| z11b_ver7.ibs * IBIS 5.0 Model
| Part Number   VDD/VDDQ   Architecture   Package
| MT40A1G8SA   1.2V/1.2V   1Gb   x 8   78-Ball FBGA
[IBIS Ver]   7.0
[File Name]   z11b_ver7.ibs
[Date]   04/03/2019
[File Rev]   1.0
[Source]   From silicon level SPICE model at Micron Technology, Inc.
[Notes]   Revision History:
   Rev 1.0: 04/03/2019
   - Initial IBIS Version 7.0 model
   - Includes Interconnect Model examples
   - Unofficial IBIS model for syntax evaluation purposes.
[Disclaimer]  This software code and all associated documentation, comments
   or other information (collectively "Software") is provided
   "AS IS" without warranty of any kind. MICRON TECHNOLOGY, INC.
   ("MTI") EXPRESSLY DISCLAIMS ALL WARRANTIES EXPRESS OR IMPLIED,
   INCLUDING BUT NOT LIMITED TO, NONINFRINGEMENT OF THIRD PARTY
   RIGHTS, AND ANY IMPLIED WARRANTIES OF MERCHANTABILITY OR
   FITNESS FOR ANY PARTICULAR PURPOSE. MTI DOES NOT WARRANT THAT
   THE SOFTWARE WILL MEET YOUR REQUIREMENTS, OR THAT THE
   OPERATION OF THE SOFTWARE WILL BE UNINTERRUPTED OR ERROR-FREE.
   FURTHERMORE, MTI DOES NOT MAKE ANY REPRESENTATIONS REGARDING
   THE USE OR THE RESULTS OF THE USE OF THE SOFTWARE IN TERMS OF
   ITS CORRECTNESS, ACCURACY, RELIABILITY, OR OTHERWISE. THE
   ENTIRE RISK ARISING OUT OF USE OR PERFORMANCE OF THE SOFTWARE
   REMAINS WITH YOU. IN NO EVENT SHALL MTI, ITS AFFILIATED
   COMPANIES OR THEIR SUPPLIERS BE LIABLE FOR ANY DIRECT,
   INDIRECT, CONSEQUENTIAL, INCIDENTAL, OR SPECIAL DAMAGES
   (INCLUDING, WITHOUT LIMITATION, DAMAGES FOR LOSS OF PROFITS,
   BUSINESS INTERRUPTION, OR LOSS OF INFORMATION) ARISING OUT OF
   YOUR USE OF OR INABILITY TO USE THE SOFTWARE, EVEN IF MTI HAS
   BEEN ADVISED OF THE POSSIBILITY OF SUCH DAMAGES. Because some
   jurisdictions prohibit the exclusion or limitation of
   liability for consequential or incidental damages, the above
   limitation may not apply to you.
   Additional Disclaimer:
   This IBIS model is unoffical and is provided to the IBIS Open
   Forum for the purposes of evaluating the IBIS Version 7.0
   syntax.  This model is not intended to accurately represent
   the characteristics of any official product.
[Copyright]   Copyright 2019 Micron Technology, Inc. All rights reserved.
| COMPONENT: MT40A1G8SA (78-Ball FBGA, x8)
[Component]   MT40A1G8SA
[Package Model] z11b_78ball_pkg
[Manufacturer]  Micron Technology,Inc.
[Package]
|   typ   min   max
R_pkg   0.420   0.337   0.508
L_pkg   1.872nH   1.600nH   2.256nH
C_pkg   0.503pF   0.373pF   0.869pF
[Pin]   signal_name   model_name   R_pin   L_pin   C_pin   | TD_pin(ps)   Z_pin
A1   VDD   POWER
A2   VSS   GND
A3   TDQS_c   TDQS   0.462   1.686nH   0.497pF   |  28.960   58.214
A7   DM_n_DBI_n_TDQS_t   DM_DBI_TDQS   0.471   1.769nH   0.574pF   |  31.858   55.533
A8   VSS   GND
A9   VSS   GND
B1   VPP   POWER
B2   VDDQ   POWER
B3   DQS_c   DQS   0.477   1.698nH   0.518pF   |  29.650   57.266
B7   DQ1   DQ   0.462   1.634nH   0.572pF   |  30.578   53.451
B8   VDDQ   POWER
B9   ZQ   NC   0.508   2.256nH   0.824pF   |  43.107   52.342
C1   VDDQ   POWER
C2   DQ0   DQ   0.462   1.655nH   0.561pF   |  30.473   54.297
C3   DQS_t   DQS   0.474   1.833nH   0.464pF   |  29.170   62.828
C7   VDD   POWER
C8   VSS   GND
C9   VDDQ   POWER
D1   VSS   GND
D2   DQ4   DQ   0.480   1.664nH   0.568pF   |  30.747   54.122
D3   DQ2   DQ   0.467   1.763nH   0.499pF   |  29.645   59.463
D7   DQ3   DQ   0.459   1.706nH   0.562pF   |  30.957   55.111
D8   DQ5   DQ   0.462   1.600nH   0.541pF   |  29.424   54.382
D9   VSS   GND
E1   VSSL   GND
E2   VDDQ   POWER
E3   DQ6   DQ   0.464   1.695nH   0.554pF   |  30.652   55.303
E7   DQ7   DQ   0.467   1.715nH   0.555pF   |  30.855   55.582
E8   VDDQ   POWER
E9   VSS   GND
F1   VDDL   POWER
F2   NC   NC
F3   ODT   INPUT   0.416   2.081nH   0.465pF   |  31.112   66.890
F7   CK_t   CLKIN   0.415   1.748nH   0.464pF   |  28.489   61.372
F8   CK_c   CLKIN   0.410   1.679nH   0.519pF   |  29.522   56.862
F9   VDD   POWER
G1   VSS   GND
G2   NC   NC
G3   CKE   INPUT   0.408   2.148nH   0.421pF   |  30.082   71.417
G7   CS_n   INPUT   0.410   1.936nH   0.441pF   |  29.202   66.289
G8   NC   NC
G9   TEN   TEN   0.391   2.104nH   0.869pF   |  42.760   49.210
H1   VDD   POWER
H2   WE_n_A14   INPUT   0.399   2.037nH   0.466pF   |  30.823   66.098
H3   ACT_n   INPUT   0.402   1.924nH   0.413pF   |  28.187   68.247
H7   CAS_n_A15   INPUT   0.400   1.971nH   0.388pF   |  27.650   71.272
H8   RAS_n   INPUT   0.402   1.982nH   0.473pF   |  30.603   64.755
H9   VSS   GND
J1   VREFCA   POWER
J2   BG0   INPUT   0.401   1.934nH   0.446pF   |  29.359   65.889
J3   A10   INPUT   0.401   1.866nH   0.389pF   |  26.938   69.285
J7   A12_BC_n   INPUT   0.399   1.954nH   0.373pF   |  26.994   72.369
J8   BG1   INPUT   0.404   2.030nH   0.462pF   |  30.632   66.264
J9   VDD   POWER
K1   VSS   GND
K2   BA0   INPUT   0.400   1.977nH   0.479pF   |  30.781   64.232
K3   A4   INPUT   0.400   1.907nH   0.431pF   |  28.681   66.498
K7   A3   INPUT   0.401   1.966nH   0.421pF   |  28.788   68.301
K8   BA1   INPUT   0.400   2.056nH   0.465pF   |  30.918   66.499
K9   VSS   GND
L1   RESET_n   RESET   0.341   1.708nH   0.725pF   |  35.193   48.541
L2   A6   INPUT   0.400   1.879nH   0.480pF   |  30.031   62.571
L3   A0   INPUT   0.401   1.714nH   0.418pF   |  26.769   64.010
L7   A1   INPUT   0.406   1.901nH   0.423pF   |  28.361   67.015
L8   A5   INPUT   0.405   1.943nH   0.492pF   |  30.910   62.868
L9   ALERT_n   ALERT   0.337   1.799nH   0.707pF   |  35.671   50.442
M1   VDD   POWER
M2   A8   INPUT   0.401   1.929nH   0.476pF   |  30.313   63.619
M3   A2   INPUT   0.403   1.906nH   0.404pF   |  27.738   68.700
M7   A9   INPUT   0.405   1.974nH   0.395pF   |  27.924   70.677
M8   A7   INPUT   0.402   2.015nH   0.488pF   |  31.361   64.239
M9   VPP   POWER
N1   VSS   GND
N2   A11   INPUT   0.401   1.858nH   0.497pF   |  30.379   61.148
N3   PARITY   INPUT   0.402   1.724nH   0.471pF   |  28.492   60.493
N7   NC   NC
N8   A13   INPUT   0.404   2.043nH   0.479pF   |  31.277   65.327
N9   VDD   POWER
|***********************PIN MAPPING*****************************************
[Pin Mapping]   pulldown_ref   pullup_ref   gnd_clamp_ref   power_clamp_ref ext_ref
A1   NC   VDD
A2   VSS   NC
A3   VSS   VDDQ   VSS   VDDQ
A7   VSS   VDDQ   VSS   VDDQ
A8   VSS   NC
A9   VSS   NC
B1   NC   VPP
B2   NC   VDDQ
B3   VSS   VDDQ   VSS   VDDQ
B7   VSS   VDDQ   VSS   VDDQ
B8   NC   VDDQ
B9   NC   NC
C1   NC   VDDQ
C2   VSS   VDDQ   VSS   VDDQ
C3   VSS   VDDQ   VSS   VDDQ
C7   NC   VDD
C8   VSS   NC
C9   NC   VDDQ
D1   VSS   NC
D2   VSS   VDDQ   VSS   VDDQ
D3   VSS   VDDQ   VSS   VDDQ
D7   VSS   VDDQ   VSS   VDDQ
D8   VSS   VDDQ   VSS   VDDQ
D9   VSS   NC
E1   VSSL   NC
E2   NC   VDDQ
E3   VSS   VDDQ   VSS   VDDQ
E7   VSS   VDDQ   VSS   VDDQ
E8   NC   VDDQ
E9   VSS   NC
F1   NC   VDDL
F2   NC   NC
F3   NC   NC   VSS   VDD
F7   NC   NC   VSS   VDD
F8   NC   NC   VSS   VDD
F9   NC   VDD
G1   VSS   NC
G2   NC   NC
G3   NC   NC   VSS   VDD
G7   NC   NC   VSS   VDD
G8   NC   NC
G9   NC   NC   VSS   VDD
H1   NC   VDD
H2   NC   NC   VSS   VDD
H3   NC   NC   VSS   VDD
H7   NC   NC   VSS   VDD
H8   NC   NC   VSS   VDD
H9   VSS   NC
J1   NC   VREFCA
J2   NC   NC   VSS   VDD
J3   NC   NC   VSS   VDD
J7   NC   NC   VSS   VDD
J8   NC   NC   VSS   VDD
J9   NC   VDD
K1   VSS   NC
K2   NC   NC   VSS   VDD
K3   NC   NC   VSS   VDD
K7   NC   NC   VSS   VDD
K8   NC   NC   VSS   VDD
K9   VSS   NC
L1   NC   NC   VSS   VDD
L2   NC   NC   VSS   VDD
L3   NC   NC   VSS   VDD
L7   NC   NC   VSS   VDD
L8   NC   NC   VSS   VDD
L9   VSS   VDDQ   VSS   VDDQ
M1   NC   VDD
M2   NC   NC   VSS   VDD
M3   NC   NC   VSS   VDD
M7   NC   NC   VSS   VDD
M8   NC   NC   VSS   VDD
M9   NC   VPP
N1   VSS   NC
N2   NC   NC   VSS   VDD
N3   NC   NC   VSS   VDD
N7   NC   NC
N8   NC   NC   VSS   VDD
N9   NC   VDD
|**********************DIE SUPPLY PADS**************************************
[Die Supply Pads]  signal_name   bus_label
VDDQ_DIE-4   VDDQ
VDDQ_DIE-8   VDDQ
VDDQ_DIE-13   VDDQ
VDDQ_DIE-16   VDDQ
VDDQ_DIE-20   VDDQ
VDDQ_DIE-25   VDDQ
VDDQ_DIE-36   VDDQ
VDDQ_DIE-48   VDDQ
VDDQ_DIE-52   VDDQ
VDDQ_DIE-62   VDDQ
VDDQ_DIE-40   VDDQ
VDDQ_DIE-45   VDDQ
VDDQ_DIE-57   VDDQ
VSS_DIE-2   VSS
VSS_DIE-6   VSS
VSS_DIE-10   VSS
VSS_DIE-11   VSS
VSS_DIE-15   VSS
VSS_DIE-18   VSS
VSS_DIE-22   VSS
VSS_DIE-23   VSS
VSS_DIE-27   VSS
VSS_DIE-28   VSS
VSS_DIE-32   VSS
VSS_DIE-34   VSS
VSS_DIE-38   VSS
VSS_DIE-42   VSS
VSS_DIE-43   VSS
VSS_DIE-47   VSS
VSS_DIE-50   VSS
VSS_DIE-54   VSS
VSS_DIE-55   VSS
VSS_DIE-59   VSS
VSS_DIE-60   VSS
VSS_DIE-64   VSS
VSS_DIE-66   VSS
VSS_DIE-69   VSS
VSS_DIE-72   VSS
VSS_DIE-93   VSS
VSS_DIE-109   VSS
VSS_DIE-117   VSS
|**********************DIFF PIN*********************************************
[Diff_pin]   inv_pin   vdiff   tdelay_typ   tdelay_min   tdelay_max
   C3   B3   0.000V   0ns   NA   NA
   F7   F8   0.250V   0ns   NA   NA
|**********************INTERCONNECT MODEL GROUPS****************************
| Interconnect Model Group for MT40A1G8SA_DQ_Signal_ISS
| Device:   MT40A1G8SA
| Signals:  DQ, DQS, DM
| Coupling: Yes
| PDN:   Ideal
| Decap:   None
| Type:   Quasi-static Spice Model
[Interconnect Model Group]  MT40A1G8SA_DQ_Signal_ISS
| Interconnect Model Set   file_reference
MT40A1G8SA_DQ_Signal_ISS   NA
[End Interconnect Model Group]
| Interconnect Model Group for MT40A1G8SA_CA_Signal_ISS
| Device:   MT40A1G8SA
| Signals:  Add, Cmd, Ctl, CLK
| Coupling: Yes
| PDN:   Ideal
| Decap:   None
| Type:   Quasi-static Spice Model
[Interconnect Model Group]  MT40A1G8SA_CA_Signal_ISS
| Interconnect Model Set   file_reference
MT40A1G8SA_CA_Signal_ISS   NA
[End Interconnect Model Group]
| Interconnect Model Group for MT40A1G8SA_Full_Pkg_ISS
| Device:   MT40A1G8SA
| Signals:  All
| Coupling: Yes
| PDN:   Package Parasitics
| Decap:   On-die
| Type:   Quasi-static Spice Model
[Interconnect Model Group]  MT40A1G8SA_Full_Pkg_ISS
| Interconnect Model Set   file_reference
MT40A1G8SA_Full_Pkg_ISS   NA
OnDie_Decoupling_AllDQ   NA
[End Interconnect Model Group]
| Interconnect Model Group for MT40A1G8SA_DQ_Signal_BB_ISS
| Device:   MT40A1G8SA
| Signals:  DQ, DQS, DM
| Coupling: Yes
| PDN:   Reference
| Decap:   None
| Type:   Full-wave Spice Model
[Interconnect Model Group]  MT40A1G8SA_DQ_Signal_BB_ISS
| Interconnect Model Set   file_reference
MT40A1G8SA_DQ_Signal_BB_ISS   NA
[End Interconnect Model Group]
| Interconnect Model Group for MT40A1G8SA_DQ_Signal_Sparam
| Device:   MT40A1G8SA
| Signals:  DQ, DQS, DM
| Coupling: Yes
| PDN:   Reference
| Decap:   None
| Type:   Full-wave S-parameter Model
[Interconnect Model Group]  MT40A1G8SA_DQ_Signal_Sparam
| Interconnect Model Set   file_reference
MT40A1G8SA_DQ_Signal_Sparam   NA
[End Interconnect Model Group]
| Interconnect Model Group for MT40A1G8SA_DQ_TS2_Sparam
| Device:   MT40A1G8SA
| Signals:  DQ, DQS, DM
| Coupling: Yes
| PDN:   Package Parasitics
| Decap:   On-die
| Type:   Full-wave S-parameter Touchstone 2.0 Model
[Interconnect Model Group]  MT40A1G8SA_DQ_TS2_Sparam
| Interconnect Model Set   file_reference
MT40A1G8SA_DQ_TS2_Sparam   NA
OnDie_Decoupling_AllDQ   NA
[End Interconnect Model Group]
| Interconnect Model Group for MT40A1G8SA_DQ_Pkg_Plus_Ondie_PDN_ISS
| Device:   MT40A1G8SA
| Signals:  DQ, DQS, DM
| Coupling: Yes
| PDN:   Package Parasitics, On-die Parasitics
| Decap:   On-die
| Type:   Quasi-static Spice Model + On-die PDN Spice Model
[Interconnect Model Group]  MT40A1G8SA_DQ_Pkg_Plus_Ondie_PDN_ISS
| Interconnect Model Set   file_reference
MT40A1G8SA_DQ_Pkg_Plus_Ondie_PDN_ISS   NA
[End Interconnect Model Group]
| Interconnect Model Group for MT40A1G8SA_DQ_Uncoupled_Sparam
| Device:   MT40A1G8SA
| Signals:  DQ, DQS, DM
| Coupling: No
| PDN:   Reference
| Decap:   On-die
| Type:   Full-wave S-parameter Models
[Interconnect Model Group]  MT40A1G8SA_DQ_Uncoupled_Sparam
| Interconnect Model Set   file_reference
MT40A1G8SA_DQ_Uncoupled_Sparam   NA
[End Interconnect Model Group]
|   Model Selector
[Model Selector] DQ
DQ_34_3200   34 Ohm Data I/O with no ODT, 1600-3200Mbps
DQ_40_3200   40 Ohm Data I/O with no ODT, 1600-3200Mbps
DQ_48_3200   48 Ohm Data I/O with no ODT, 1600-3200Mbps
DQ_IN_ODTOFF_3200  Data Input with no ODT, 1600-3200Mbps
DQ_IN_ODT34_3200   Data Input with 34ohm ODT, 1600-3200Mbps
DQ_IN_ODT40_3200   Data Input with 40ohm ODT, 1600-3200Mbps
DQ_IN_ODT48_3200   Data Input with 48ohm ODT, 1600-3200Mbps
DQ_IN_ODT60_3200   Data Input with 60ohm ODT, 1600-3200Mbps
DQ_IN_ODT80_3200   Data Input with 80ohm ODT, 1600-3200Mbps
DQ_IN_ODT120_3200  Data Input with 120ohm ODT, 1600-3200Mbps
DQ_IN_ODT240_3200  Data Input with 240ohm ODT, 1600-3200Mbps
[Model Selector] DQS
DQS_34_3200   34 Ohm Data Strobe I/O with no ODT, 1600-3200Mbps
DQS_40_3200   40 Ohm Data Strobe I/O with no ODT, 1600-3200Mbps
DQS_48_3200   48 Ohm Data Strobe I/O with no ODT, 1600-3200Mbps
DQS_IN_ODTOFF_3200 Data Strobe Input with no ODT, 1600-3200Mbps
DQS_IN_ODT34_3200  Data Strobe Input with 34ohm ODT, 1600-3200Mbps
DQS_IN_ODT40_3200  Data Strobe Input with 40ohm ODT, 1600-3200Mbps
DQS_IN_ODT48_3200  Data Strobe Input with 48ohm ODT, 1600-3200Mbps
DQS_IN_ODT60_3200  Data Strobe Input with 60ohm ODT, 1600-3200Mbps
DQS_IN_ODT80_3200  Data Strobe Input with 80ohm ODT, 1600-3200Mbps
DQS_IN_ODT120_3200 Data Strobe Input with 120ohm ODT, 1600-3200Mbps
DQS_IN_ODT240_3200 Data Strobe Input with 240ohm ODT, 1600-3200Mbps
[Model Selector] DM_DBI
DM_ODTOFF_3200   DM Input Model with no ODT, 1600-3200Mbps
DM_ODT34_3200   DM Input Model with 34ohm ODT, 1600-3200Mbps
DM_ODT40_3200   DM Input Model with 40ohm ODT, 1600-3200Mbps
DM_ODT48_3200   DM Input Model with 48ohm ODT, 1600-3200Mbps
DM_ODT60_3200   DM Input Model with 60ohm ODT, 1600-3200Mbps
DM_ODT80_3200   DM Input Model with 80ohm ODT, 1600-3200Mbps
DM_ODT120_3200   DM Input Model with 120ohm ODT, 1600-3200Mbps
DM_ODT240_3200   DM Input Model with 240ohm ODT, 1600-3200Mbps
DQ_34_3200   34 Ohm DBI I/O with no ODT, 1600-3200Mbps
DQ_40_3200   40 Ohm DBI I/O with no ODT, 1600-3200Mbps
DQ_48_3200   48 Ohm DBI I/O with no ODT, 1600-3200Mbps
DQ_IN_ODTOFF_3200  DBI Input with no ODT, 1600-3200Mbps
DQ_IN_ODT34_3200   DBI Input with 34ohm ODT, 1600-3200Mbps
DQ_IN_ODT40_3200   DBI Input with 40ohm ODT, 1600-3200Mbps
DQ_IN_ODT48_3200   DBI Input with 48ohm ODT, 1600-3200Mbps
DQ_IN_ODT60_3200   DBI Input with 60ohm ODT, 1600-3200Mbps
DQ_IN_ODT80_3200   DBI Input with 80ohm ODT, 1600-3200Mbps
DQ_IN_ODT120_3200  DBI Input with 120ohm ODT, 1600-3200Mbps
DQ_IN_ODT240_3200  DBI Input with 240ohm ODT, 1600-3200Mbps
NF_DQ   Non-Functioning DQ Terminator Model
[Model Selector] DM_DBI_TDQS
DM_ODTOFF_3200   DM Input Model with no ODT, 1600-3200Mbps
DM_ODT34_3200   DM Input Model with 34ohm ODT, 1600-3200Mbps
DM_ODT40_3200   DM Input Model with 40ohm ODT, 1600-3200Mbps
DM_ODT48_3200   DM Input Model with 48ohm ODT, 1600-3200Mbps
DM_ODT60_3200   DM Input Model with 60ohm ODT, 1600-3200Mbps
DM_ODT80_3200   DM Input Model with 80ohm ODT, 1600-3200Mbps
DM_ODT120_3200   DM Input Model with 120ohm ODT, 1600-3200Mbps
DM_ODT240_3200   DM Input Model with 240ohm ODT, 1600-3200Mbps
DQ_34_3200   34 Ohm DBI I/O with no ODT, 1600-3200Mbps
DQ_40_3200   40 Ohm DBI I/O with no ODT, 1600-3200Mbps
DQ_48_3200   48 Ohm DBI I/O with no ODT, 1600-3200Mbps
DQ_IN_ODTOFF_3200  DBI Input with no ODT, 1600-3200Mbps
DQ_IN_ODT34_3200   DBI Input with 34ohm ODT, 1600-3200Mbps
DQ_IN_ODT40_3200   DBI Input with 40ohm ODT, 1600-3200Mbps
DQ_IN_ODT48_3200   DBI Input with 48ohm ODT, 1600-3200Mbps
DQ_IN_ODT60_3200   DBI Input with 60ohm ODT, 1600-3200Mbps
DQ_IN_ODT80_3200   DBI Input with 80ohm ODT, 1600-3200Mbps
DQ_IN_ODT120_3200  DBI Input with 120ohm ODT, 1600-3200Mbps
DQ_IN_ODT240_3200  DBI Input with 240ohm ODT, 1600-3200Mbps
TDQS_ODTOFF_3200   TDQS Terminator Model with no ODT, 1600-3200Mbps
TDQS_ODT34_3200   TDQS Terminator Model with 34ohm ODT, 1600-3200Mbps
TDQS_ODT40_3200   TDQS Terminator Model with 40ohm ODT, 1600-3200Mbps
TDQS_ODT48_3200   TDQS Terminator Model with 48ohm ODT, 1600-3200Mbps
TDQS_ODT60_3200   TDQS Terminator Model with 60ohm ODT, 1600-3200Mbps
TDQS_ODT80_3200   TDQS Terminator Model with 80ohm ODT, 1600-3200Mbps
TDQS_ODT120_3200   TDQS Terminator Model with 120ohm ODT, 1600-3200Mbps
TDQS_ODT240_3200   TDQS Terminator Model with 240ohm ODT, 1600-3200Mbps
NF_DQ   Non-Functioning DQ Terminator Model
[Model Selector] TDQS
TDQS_ODTOFF_3200   TDQS Terminator Model with no ODT, 1600-3200Mbps
TDQS_ODT34_3200   TDQS Terminator Model with 34ohm ODT, 1600-3200Mbps
TDQS_ODT40_3200   TDQS Terminator Model with 40ohm ODT, 1600-3200Mbps
TDQS_ODT48_3200   TDQS Terminator Model with 48ohm ODT, 1600-3200Mbps
TDQS_ODT60_3200   TDQS Terminator Model with 60ohm ODT, 1600-3200Mbps
TDQS_ODT80_3200   TDQS Terminator Model with 80ohm ODT, 1600-3200Mbps
TDQS_ODT120_3200   TDQS Terminator Model with 120ohm ODT, 1600-3200Mbps
TDQS_ODT240_3200   TDQS Terminator Model with 240ohm ODT, 1600-3200Mbps
NF_DQ   Non-Functioning DQ Terminator Model
| Sparse Matrix Package Model for z11b_78ball_pkg (x4/x8)
[Define Package Model]  z11b_78ball_pkg
[Manufacturer]   Micron Technology, Inc.
[OEM]   Micron Technology, Inc.
[Description]   z11b package model for 78-ball x4/x8 FBGA
[Number of Pins]   51
[Pin Numbers]
L3  | A0
L7  | A1
M3  | A2
K7  | A3
K3  | A4
L8  | A5
L2  | A6
M8  | A7
M2  | A8
M7  | A9
J3  | A10
N2  | A11
J7  | A12
N8  | A13
H3  | ACT#
L9  | ALERT#
K2  | BA0
K8  | BA1
J2  | BG0
J8  | BG1
H7  | CAS#
G3  | CKE
F8  | CK_C
F7  | CK_T
G7  | CS#
F3  | ODT
N3  | PARITY
H8  | RAS#
L1  | RESET#
H2  | WE#
C2  | DQ0
D3  | DQ2
D2  | DQ4
E3  | DQ6
B3  | DQS-C
C3  | DQS-T
A3  | TDQS-C
A7  | DM#
B7  | DQ1
D7  | DQ3
D8  | DQ5
E7  | DQ7
G9  | TEN
A1  | VDD
B2  | VDDQ_SUBNET_0
B8  | VDDQ_SUBNET_1
B1  | VPP-B1
M9  | VPP-M9
J1  | VREFCA
A9  | VSS
B9  | ZQ
[Model Data]
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[End Model Data]
[End Package Model]
| Interconnect Model Set for MT40A1G8SA_DQ_Signal_ISS
[Interconnect Model Set]   MT40A1G8SA_DQ_Signal_ISS
[Manufacturer]   Micron Technology, Inc.
[Description]   Z11B 78b, DQ signal only, Coupled Spice Package Model
[Interconnect Model]   z11b_78b_pkg_dq_iss
File_IBIS-ISS   z11b_78b_pkg_dq.iss   z11b_rlc_dq_pkg
Number_of_terminals = 25
1   Buffer_I/O   pin_name   A7   |   DM_n_DBI_n_TDQS_t  DM_DBI_TDQS
2   Buffer_I/O   pin_name   C2   |   DQ0   DQ
3   Buffer_I/O   pin_name   B7   |   DQ1   DQ
4   Buffer_I/O   pin_name   D3   |   DQ2   DQ
5   Buffer_I/O   pin_name   D7   |   DQ3   DQ
6   Buffer_I/O   pin_name   D2   |   DQ4   DQ
7   Buffer_I/O   pin_name   D8   |   DQ5   DQ
8   Buffer_I/O   pin_name   E3   |   DQ6   DQ
9   Buffer_I/O   pin_name   E7   |   DQ7   DQ
10   Buffer_I/O   pin_name   B3   |   DQS_c   DQS
11   Buffer_I/O   pin_name   C3   |   DQS_t   DQS
12   Buffer_I/O   pin_name   A3   |   TDQS_c   TDQS
13   Pin_I/O   pin_name   A7   |   DM_n_DBI_n_TDQS_t  DM_DBI_TDQS
14   Pin_I/O   pin_name   C2   |   DQ0   DQ
15   Pin_I/O   pin_name   B7   |   DQ1   DQ
16   Pin_I/O   pin_name   D3   |   DQ2   DQ
17   Pin_I/O   pin_name   D7   |   DQ3   DQ
18   Pin_I/O   pin_name   D2   |   DQ4   DQ
19   Pin_I/O   pin_name   D8   |   DQ5   DQ
20   Pin_I/O   pin_name   E3   |   DQ6   DQ
21   Pin_I/O   pin_name   E7   |   DQ7   DQ
22   Pin_I/O   pin_name   B3   |   DQS_c   DQS
23   Pin_I/O   pin_name   C3   |   DQS_t   DQS
24   Pin_I/O   pin_name   A3   |   TDQS_c   TDQS
25   Pin_Rail   signal_name   VSS   |   VSS   GND
[End Interconnect Model]
[End Interconnect Model Set]
| Interconnect Model Set for MT40A1G8SA_CA_Signal_ISS
[Interconnect Model Set]   MT40A1G8SA_CA_Signal_ISS
[Manufacturer]   Micron Technology, Inc.
[Description]   Z11B 78b, CA signal only, Coupled Spice Package Model
[Interconnect Model]   z11b_78b_pkg_ca_iss
File_IBIS-ISS   z11b_78b_pkg_ca.iss   z11b_rlc_ca_pkg
Number_of_terminals = 63
1   Buffer_I/O   pin_name   L3   |   A0   INPUT
2   Buffer_I/O   pin_name   L7   |   A1   INPUT
3   Buffer_I/O   pin_name   M3   |   A2   INPUT
4   Buffer_I/O   pin_name   K7   |   A3   INPUT
5   Buffer_I/O   pin_name   K3   |   A4   INPUT
6   Buffer_I/O   pin_name   L8   |   A5   INPUT
7   Buffer_I/O   pin_name   L2   |   A6   INPUT
8   Buffer_I/O   pin_name   M8   |   A7   INPUT
9   Buffer_I/O   pin_name   M2   |   A8   INPUT
10   Buffer_I/O   pin_name   M7   |   A9   INPUT
11   Buffer_I/O   pin_name   J3   |   A10   INPUT
12   Buffer_I/O   pin_name   N2   |   A11   INPUT
13   Buffer_I/O   pin_name   J7   |   A12_BC_n   INPUT
14   Buffer_I/O   pin_name   N8   |   A13   INPUT
15   Buffer_I/O   pin_name   H3   |   ACT_n   INPUT
16   Buffer_I/O   pin_name   L9   |   ALERT_n   ALERT
17   Buffer_I/O   pin_name   K2   |   BA0   INPUT
18   Buffer_I/O   pin_name   K8   |   BA1   INPUT
19   Buffer_I/O   pin_name   J2   |   BG0   INPUT
20   Buffer_I/O   pin_name   J8   |   BG1   INPUT
21   Buffer_I/O   pin_name   H7   |   CAS_n_A15   INPUT
22   Buffer_I/O   pin_name   G3   |   CKE   INPUT
23   Buffer_I/O   pin_name   F8   |   CK_c   CLKIN
24   Buffer_I/O   pin_name   F7   |   CK_t   CLKIN
25   Buffer_I/O   pin_name   G7   |   CS_n   INPUT
26   Buffer_I/O   pin_name   N3   |   PARITY   INPUT
27   Buffer_I/O   pin_name   H8   |   RAS_n   INPUT
28   Buffer_I/O   pin_name   L1   |   RESET_n   RESET
29   Buffer_I/O   pin_name   G9   |   TEN   TEN
30   Buffer_Rail   bus_label   VREFCA  |   VREFCA   POWER
31   Buffer_I/O   pin_name   H2   |   WE_n_A14   INPUT
32   Pin_I/O   pin_name   L3   |   A0   INPUT
33   Pin_I/O   pin_name   L7   |   A1   INPUT
34   Pin_I/O   pin_name   M3   |   A2   INPUT
35   Pin_I/O   pin_name   K7   |   A3   INPUT
36   Pin_I/O   pin_name   K3   |   A4   INPUT
37   Pin_I/O   pin_name   L8   |   A5   INPUT
38   Pin_I/O   pin_name   L2   |   A6   INPUT
39   Pin_I/O   pin_name   M8   |   A7   INPUT
40   Pin_I/O   pin_name   M2   |   A8   INPUT
41   Pin_I/O   pin_name   M7   |   A9   INPUT
42   Pin_I/O   pin_name   J3   |   A10   INPUT
43   Pin_I/O   pin_name   N2   |   A11   INPUT
44   Pin_I/O   pin_name   J7   |   A12_BC_n   INPUT
45   Pin_I/O   pin_name   N8   |   A13   INPUT
46   Pin_I/O   pin_name   H3   |   ACT_n   INPUT
47   Pin_I/O   pin_name   L9   |   ALERT_n   ALERT
48   Pin_I/O   pin_name   K2   |   BA0   INPUT
49   Pin_I/O   pin_name   K8   |   BA1   INPUT
50   Pin_I/O   pin_name   J2   |   BG0   INPUT
51   Pin_I/O   pin_name   J8   |   BG1   INPUT
52   Pin_I/O   pin_name   H7   |   CAS_n_A15   INPUT
53   Pin_I/O   pin_name   G3   |   CKE   INPUT
54   Pin_I/O   pin_name   F8   |   CK_c   CLKIN
55   Pin_I/O   pin_name   F7   |   CK_t   CLKIN
56   Pin_I/O   pin_name   G7   |   CS_n   INPUT
57   Pin_I/O   pin_name   N3   |   PARITY   INPUT
58   Pin_I/O   pin_name   H8   |   RAS_n   INPUT
59   Pin_I/O   pin_name   L1   |   RESET_n   RESET
60   Pin_I/O   pin_name   G9   |   TEN   TEN
61   Pin_Rail   pin_name   J1   |   VREFCA   POWER
62   Pin_I/O   pin_name   H2   |   WE_n_A14   INPUT
63   Pin_Rail   signal_name   VSS   |   VSS   GND
[End Interconnect Model]
[End Interconnect Model Set]
| Interconnect Model Set for MT40A1G8SA_Full_Pkg_ISS
[Interconnect Model Set]   MT40A1G8SA_Full_Pkg_ISS
[Manufacturer]   Micron Technology, Inc.
[Description]   Z11B 78b, Full Package, Coupled Spice Model
[Interconnect Model]   z11b_78b_full_pkg_iss
File_IBIS-ISS   z11b_78b_full_pkg.iss   z11b_rlc_all_pkg
Number_of_terminals = 104
1   Buffer_I/O   pin_name   L3   |   A0   INPUT
2   Buffer_I/O   pin_name   L7   |   A1   INPUT
3   Buffer_I/O   pin_name   M3   |   A2   INPUT
4   Buffer_I/O   pin_name   K7   |   A3   INPUT
5   Buffer_I/O   pin_name   K3   |   A4   INPUT
6   Buffer_I/O   pin_name   L8   |   A5   INPUT
7   Buffer_I/O   pin_name   L2   |   A6   INPUT
8   Buffer_I/O   pin_name   M8   |   A7   INPUT
9   Buffer_I/O   pin_name   M2   |   A8   INPUT
10   Buffer_I/O   pin_name   M7   |   A9   INPUT
11   Buffer_I/O   pin_name   J3   |   A10   INPUT
12   Buffer_I/O   pin_name   N2   |   A11   INPUT
13   Buffer_I/O   pin_name   J7   |   A12_BC_n   INPUT
14   Buffer_I/O   pin_name   N8   |   A13   INPUT
15   Buffer_I/O   pin_name   H3   |   ACT_n   INPUT
16   Buffer_I/O   pin_name   L9   |   ALERT_n   ALERT
17   Buffer_I/O   pin_name   K2   |   BA0   INPUT
18   Buffer_I/O   pin_name   K8   |   BA1   INPUT
19   Buffer_I/O   pin_name   J2   |   BG0   INPUT
20   Buffer_I/O   pin_name   J8   |   BG1   INPUT
21   Buffer_I/O   pin_name   H7   |   CAS_n_A15   INPUT
22   Buffer_I/O   pin_name   G3   |   CKE   INPUT
23   Buffer_I/O   pin_name   F8   |   CK_c   CLKIN
24   Buffer_I/O   pin_name   F7   |   CK_t   CLKIN
25   Buffer_I/O   pin_name   G7   |   CS_n   INPUT
26   Buffer_I/O   pin_name   A7   |   DM_n_DBI_n_TDQS_t  DM_DBI_TDQS
27   Buffer_I/O   pin_name   C2   |   DQ0   DQ
28   Buffer_I/O   pin_name   B7   |   DQ1   DQ
29   Buffer_I/O   pin_name   D3   |   DQ2   DQ
30   Buffer_I/O   pin_name   D7   |   DQ3   DQ
31   Buffer_I/O   pin_name   D2   |   DQ4   DQ
32   Buffer_I/O   pin_name   D8   |   DQ5   DQ
33   Buffer_I/O   pin_name   E3   |   DQ6   DQ
34   Buffer_I/O   pin_name   E7   |   DQ7   DQ
35   Buffer_I/O   pin_name   B3   |   DQS_c   DQS
36   Buffer_I/O   pin_name   C3   |   DQS_t   DQS
37   Buffer_I/O   pin_name   F3   |   ODT   INPUT
38   Buffer_I/O   pin_name   N3   |   PARITY   INPUT
39   Buffer_I/O   pin_name   H8   |   RAS_n   INPUT
40   Buffer_I/O   pin_name   L1   |   RESET_n   RESET
41   Buffer_I/O   pin_name   A3   |   TDQS_c   TDQS
42   Buffer_I/O   pin_name   G9   |   TEN   TEN
43   Buffer_Rail   bus_label   VDD   |   VDD   POWER
44   Buffer_Rail   bus_label   VDDL   |   VDDL   POWER
45   Buffer_Rail   bus_label   VDDQ   |   VDDQ   POWER
46   Buffer_Rail   bus_label   VDDQ   |   VDDQ   POWER
47   Buffer_Rail   bus_label   VPP   |   VPP   POWER
48   Buffer_Rail   bus_label   VPP   |   VPP   POWER
49   Buffer_Rail   bus_label   VREFCA  |   VREFCA   POWER
50   Buffer_Rail   bus_label   VSS   |   VSS   GND
51   Buffer_I/O   pin_name   H2   |   WE_n_A14   INPUT
52   Buffer_I/O   pin_name   B9   |   ZQ   NC
53   Pin_I/O   pin_name   L3   |   A0   INPUT
54   Pin_I/O   pin_name   L7   |   A1   INPUT
55   Pin_I/O   pin_name   M3   |   A2   INPUT
56   Pin_I/O   pin_name   K7   |   A3   INPUT
57   Pin_I/O   pin_name   K3   |   A4   INPUT
58   Pin_I/O   pin_name   L8   |   A5   INPUT
59   Pin_I/O   pin_name   L2   |   A6   INPUT
60   Pin_I/O   pin_name   M8   |   A7   INPUT
61   Pin_I/O   pin_name   M2   |   A8   INPUT
62   Pin_I/O   pin_name   M7   |   A9   INPUT
63   Pin_I/O   pin_name   J3   |   A10   INPUT
64   Pin_I/O   pin_name   N2   |   A11   INPUT
65   Pin_I/O   pin_name   J7   |   A12_BC_n   INPUT
66   Pin_I/O   pin_name   N8   |   A13   INPUT
67   Pin_I/O   pin_name   H3   |   ACT_n   INPUT
68   Pin_I/O   pin_name   L9   |   ALERT_n   ALERT
69   Pin_I/O   pin_name   K2   |   BA0   INPUT
70   Pin_I/O   pin_name   K8   |   BA1   INPUT
71   Pin_I/O   pin_name   J2   |   BG0   INPUT
72   Pin_I/O   pin_name   J8   |   BG1   INPUT
73   Pin_I/O   pin_name   H7   |   CAS_n_A15   INPUT
74   Pin_I/O   pin_name   G3   |   CKE   INPUT
75   Pin_I/O   pin_name   F8   |   CK_c   CLKIN
76   Pin_I/O   pin_name   F7   |   CK_t   CLKIN
77   Pin_I/O   pin_name   G7   |   CS_n   INPUT
78   Pin_I/O   pin_name   A7   |   DM_n_DBI_n_TDQS_t  DM_DBI_TDQS
79   Pin_I/O   pin_name   C2   |   DQ0   DQ
80   Pin_I/O   pin_name   B7   |   DQ1   DQ
81   Pin_I/O   pin_name   D3   |   DQ2   DQ
82   Pin_I/O   pin_name   D7   |   DQ3   DQ
83   Pin_I/O   pin_name   D2   |   DQ4   DQ
84   Pin_I/O   pin_name   D8   |   DQ5   DQ
85   Pin_I/O   pin_name   E3   |   DQ6   DQ
86   Pin_I/O   pin_name   E7   |   DQ7   DQ
87   Pin_I/O   pin_name   B3   |   DQS_c   DQS
88   Pin_I/O   pin_name   C3   |   DQS_t   DQS
89   Pin_I/O   pin_name   F3   |   ODT   INPUT
90   Pin_I/O   pin_name   N3   |   PARITY   INPUT
91   Pin_I/O   pin_name   H8   |   RAS_n   INPUT
92   Pin_I/O   pin_name   L1   |   RESET_n   RESET
93   Pin_I/O   pin_name   A3   |   TDQS_c   TDQS
94   Pin_I/O   pin_name   G9   |   TEN   TEN
95   Pin_Rail   pin_name   A1   |   VDD   POWER
96   Pin_Rail   pin_name   F1   |   VDDL   POWER
97   Pin_Rail   pin_name   B2   |   VDDQ   POWER
98   Pin_Rail   pin_name   C9   |   VDDQ   POWER
99   Pin_Rail   pin_name   B1   |   VPP   POWER
100   Pin_Rail   pin_name   M9   |   VPP   POWER
101   Pin_Rail   pin_name   J1   |   VREFCA   POWER
102   Pin_Rail   pin_name   A9   |   VSS   GND
103   Pin_I/O   pin_name   H2   |   WE_n_A14   INPUT
104   Pin_I/O   pin_name   B9   |   ZQ   NC
[End Interconnect Model]
[End Interconnect Model Set]
| Interconnect Model Set for OnDie_Decoupling_AllDQ
[Interconnect Model Set]   OnDie_Decoupling_AllDQ
[Interconnect Model]   z11b_ondie_decoupling_alldq_iss
File_IBIS-ISS   z11b_ondie_decoupling_alldq.iss   z11b_ondie_decoupling_alldq
Number_of_terminals = 4
1   Buffer_Rail   bus_label   VDDQ   |   VDDQ   POWER
2   Buffer_Rail   bus_label   VDD   |   VDD   POWER
3   Buffer_Rail   bus_label   VSS   |   VSS   GND
4   A_gnd
[End Interconnect Model]
[End Interconnect Model Set]
| Interconnect Model Set for MT40A1G8SA_DQ_Signal_BB_ISS
[Interconnect Model Set]   MT40A1G8SA_DQ_Signal_BB_ISS
[Interconnect Model]   z11b_78b_bb_dq_pkg_iss
File_IBIS-ISS   z11b_78b_bb_dq_pkg.iss   z11b_bb_dq_pkg
Number_of_terminals = 25
1   Pin_I/O   pin_name   A7   |   DM_n_DBI_n_TDQS_t  DM_DBI_TDQS
2   Buffer_I/O   pin_name   A7   |   DM_n_DBI_n_TDQS_t  DM_DBI_TDQS
3   Pin_I/O   pin_name   C2   |   DQ0   DQ
4   Buffer_I/O   pin_name   C2   |   DQ0   DQ
5   Pin_I/O   pin_name   B7   |   DQ1   DQ
6   Buffer_I/O   pin_name   B7   |   DQ1   DQ
7   Pin_I/O   pin_name   D3   |   DQ2   DQ
8   Buffer_I/O   pin_name   D3   |   DQ2   DQ
9   Pin_I/O   pin_name   D7   |   DQ3   DQ
10   Buffer_I/O   pin_name   D7   |   DQ3   DQ
11   Pin_I/O   pin_name   D2   |   DQ4   DQ
12   Buffer_I/O   pin_name   D2   |   DQ4   DQ
13   Pin_I/O   pin_name   D8   |   DQ5   DQ
14   Buffer_I/O   pin_name   D8   |   DQ5   DQ
15   Pin_I/O   pin_name   E3   |   DQ6   DQ
16   Buffer_I/O   pin_name   E3   |   DQ6   DQ
17   Pin_I/O   pin_name   E7   |   DQ7   DQ
18   Buffer_I/O   pin_name   E7   |   DQ7   DQ
19   Pin_I/O   pin_name   B3   |   DQS_c   DQS
20   Buffer_I/O   pin_name   B3   |   DQS_c   DQS
21   Pin_I/O   pin_name   C3   |   DQS_t   DQS
22   Buffer_I/O   pin_name   C3   |   DQS_t   DQS
23   Pin_I/O   pin_name   A3   |   TDQS_c   TDQS
24   Buffer_I/O   pin_name   A3   |   TDQS_c   TDQS
25   Pin_Rail   signal_name   VSS   |   VSS   GND
[End Interconnect Model]
[End Interconnect Model Set]
| Interconnect Model Set for MT40A1G8SA_DQ_Signal_Sparam
[Interconnect Model Set]   MT40A1G8SA_DQ_Signal_Sparam
[Interconnect Model]   z11b_78b_dq_sparam_s24p
File_TS   z11b_78b_dq_sparam.s24p
Number_of_terminals = 25
1   Pin_I/O   pin_name   A7   |   DM_n_DBI_n_TDQS_t  DM_DBI_TDQS
2   Buffer_I/O   pin_name   A7   |   DM_n_DBI_n_TDQS_t  DM_DBI_TDQS
3   Pin_I/O   pin_name   C2   |   DQ0   DQ
4   Buffer_I/O   pin_name   C2   |   DQ0   DQ
5   Pin_I/O   pin_name   B7   |   DQ1   DQ
6   Buffer_I/O   pin_name   B7   |   DQ1   DQ
7   Pin_I/O   pin_name   D3   |   DQ2   DQ
8   Buffer_I/O   pin_name   D3   |   DQ2   DQ
9   Pin_I/O   pin_name   D7   |   DQ3   DQ
10   Buffer_I/O   pin_name   D7   |   DQ3   DQ
11   Pin_I/O   pin_name   D2   |   DQ4   DQ
12   Buffer_I/O   pin_name   D2   |   DQ4   DQ
13   Pin_I/O   pin_name   D8   |   DQ5   DQ
14   Buffer_I/O   pin_name   D8   |   DQ5   DQ
15   Pin_I/O   pin_name   E3   |   DQ6   DQ
16   Buffer_I/O   pin_name   E3   |   DQ6   DQ
17   Pin_I/O   pin_name   E7   |   DQ7   DQ
18   Buffer_I/O   pin_name   E7   |   DQ7   DQ
19   Pin_I/O   pin_name   B3   |   DQS_c   DQS
20   Buffer_I/O   pin_name   B3   |   DQS_c   DQS
21   Pin_I/O   pin_name   C3   |   DQS_t   DQS
22   Buffer_I/O   pin_name   C3   |   DQS_t   DQS
23   Pin_I/O   pin_name   A3   |   TDQS_c   TDQS
24   Buffer_I/O   pin_name   A3   |   TDQS_c   TDQS
25   Pin_Rail   signal_name   VSS   |   VSS   GND
[End Interconnect Model]
[End Interconnect Model Set]
| Interconnect Model Set for MT40A1G8SA_DQ_TS2_Sparam
[Interconnect Model Set]   MT40A1G8SA_DQ_TS2_Sparam
[Interconnect Model]   z11b_78b_dq_ts2_s28p
File_TS   z11b_78b_dq_ts2.s28p
Number_of_terminals = 29
1   Pin_I/O   pin_name   A7   |   DM_n_DBI_n_TDQS_t  DM_DBI_TDQS
2   Buffer_I/O   pin_name   A7   |   DM_n_DBI_n_TDQS_t  DM_DBI_TDQS
3   Pin_I/O   pin_name   C2   |   DQ0   DQ
4   Buffer_I/O   pin_name   C2   |   DQ0   DQ
5   Pin_I/O   pin_name   B7   |   DQ1   DQ
6   Buffer_I/O   pin_name   B7   |   DQ1   DQ
7   Pin_I/O   pin_name   D3   |   DQ2   DQ
8   Buffer_I/O   pin_name   D3   |   DQ2   DQ
9   Pin_I/O   pin_name   D7   |   DQ3   DQ
10   Buffer_I/O   pin_name   D7   |   DQ3   DQ
11   Pin_I/O   pin_name   D2   |   DQ4   DQ
12   Buffer_I/O   pin_name   D2   |   DQ4   DQ
13   Pin_I/O   pin_name   D8   |   DQ5   DQ
14   Buffer_I/O   pin_name   D8   |   DQ5   DQ
15   Pin_I/O   pin_name   E3   |   DQ6   DQ
16   Buffer_I/O   pin_name   E3   |   DQ6   DQ
17   Pin_I/O   pin_name   E7   |   DQ7   DQ
18   Buffer_I/O   pin_name   E7   |   DQ7   DQ
19   Pin_I/O   pin_name   B3   |   DQS_c   DQS
20   Buffer_I/O   pin_name   B3   |   DQS_c   DQS
21   Pin_I/O   pin_name   C3   |   DQS_t   DQS
22   Buffer_I/O   pin_name   C3   |   DQS_t   DQS
23   Pin_Rail   pin_name   A1   |   VDD   POWER
24   Buffer_Rail   bus_label   VDD   |   VDD   POWER
25   Pin_Rail   pin_name   B2   |   VDDQ   POWER
26   Buffer_Rail   bus_label   VDDQ   |   VDDQ   POWER
27   Pin_Rail   pin_name   B8   |   VDDQ   POWER
28   Buffer_Rail   bus_label   VDDQ   |   VDDQ   POWER
29   Pin_Rail   signal_name   VSS   |   VSS   GND
[End Interconnect Model]
[End Interconnect Model Set]
| Interconnect Model Set for MT40A1G8SA_DQ_Pkg_Plus_Ondie_PDN_ISS
[Interconnect Model Set]   MT40A1G8SA_DQ_Pkg_Plus_Ondie_PDN_ISS
[Interconnect Model]   Z11B_78b_DQ_unmerged_pkg_iss
File_IBIS-ISS   z11b_78b_DQ_unmerged.iss   Z11B_78b_DQ_unmerged_rlc
Number_of_terminals = 67
1   Pad_I/O   pin_name   A7   |   DM_n_DBI_n_TDQS_t  DM_DBI_TDQS
2   Pad_I/O   pin_name   C2   |   DQ0   DQ
3   Pad_I/O   pin_name   B7   |   DQ1   DQ
4   Pad_I/O   pin_name   D3   |   DQ2   DQ
5   Pad_I/O   pin_name   D7   |   DQ3   DQ
6   Pad_I/O   pin_name   D2   |   DQ4   DQ
7   Pad_I/O   pin_name   D8   |   DQ5   DQ
8   Pad_I/O   pin_name   E3   |   DQ6   DQ
9   Pad_I/O   pin_name   E7   |   DQ7   DQ
10   Pad_I/O   pin_name   B3   |   DQS_c   DQS
11   Pad_I/O   pin_name   C3   |   DQS_t   DQS
12   Pad_Rail   pad_name   VDDQ_DIE-4   |   VDDQ   POWER
13   Pad_Rail   pad_name   VDDQ_DIE-8   |   VDDQ   POWER
14   Pad_Rail   pad_name   VDDQ_DIE-13  |   VDDQ   POWER
15   Pad_Rail   pad_name   VDDQ_DIE-16  |   VDDQ   POWER
16   Pad_Rail   pad_name   VDDQ_DIE-20  |   VDDQ   POWER
17   Pad_Rail   pad_name   VDDQ_DIE-25  |   VDDQ   POWER
18   Pad_Rail   pad_name   VDDQ_DIE-36  |   VDDQ   POWER
19   Pad_Rail   pad_name   VDDQ_DIE-48  |   VDDQ   POWER
20   Pad_Rail   pad_name   VDDQ_DIE-52  |   VDDQ   POWER
21   Pad_Rail   pad_name   VDDQ_DIE-62  |   VDDQ   POWER
22   Pad_Rail   pad_name   VDDQ_DIE-40  |   VDDQ   POWER
23   Pad_Rail   pad_name   VDDQ_DIE-45  |   VDDQ   POWER
24   Pad_Rail   pad_name   VDDQ_DIE-57  |   VDDQ   POWER
25   Pad_Rail   pad_name   VSS_DIE-2   |   VSS   GND
26   Pad_Rail   pad_name   VSS_DIE-6   |   VSS   GND
27   Pad_Rail   pad_name   VSS_DIE-10   |   VSS   GND
28   Pad_Rail   pad_name   VSS_DIE-11   |   VSS   GND
29   Pad_Rail   pad_name   VSS_DIE-15   |   VSS   GND
30   Pad_Rail   pad_name   VSS_DIE-18   |   VSS   GND
31   Pad_Rail   pad_name   VSS_DIE-22   |   VSS   GND
32   Pad_Rail   pad_name   VSS_DIE-23   |   VSS   GND
33   Pad_Rail   pad_name   VSS_DIE-27   |   VSS   GND
34   Pad_Rail   pad_name   VSS_DIE-28   |   VSS   GND
35   Pad_Rail   pad_name   VSS_DIE-32   |   VSS   GND
36   Pad_Rail   pad_name   VSS_DIE-34   |   VSS   GND
37   Pad_Rail   pad_name   VSS_DIE-38   |   VSS   GND
38   Pad_Rail   pad_name   VSS_DIE-42   |   VSS   GND
39   Pad_Rail   pad_name   VSS_DIE-43   |   VSS   GND
40   Pad_Rail   pad_name   VSS_DIE-47   |   VSS   GND
41   Pad_Rail   pad_name   VSS_DIE-50   |   VSS   GND
42   Pad_Rail   pad_name   VSS_DIE-54   |   VSS   GND
43   Pad_Rail   pad_name   VSS_DIE-55   |   VSS   GND
44   Pad_Rail   pad_name   VSS_DIE-59   |   VSS   GND
45   Pad_Rail   pad_name   VSS_DIE-60   |   VSS   GND
46   Pad_Rail   pad_name   VSS_DIE-64   |   VSS   GND
47   Pad_Rail   pad_name   VSS_DIE-66   |   VSS   GND
48   Pad_Rail   pad_name   VSS_DIE-69   |   VSS   GND
49   Pad_Rail   pad_name   VSS_DIE-72   |   VSS   GND
50   Pad_Rail   pad_name   VSS_DIE-93   |   VSS   GND
51   Pad_Rail   pad_name   VSS_DIE-109  |   VSS   GND
52   Pad_Rail   pad_name   VSS_DIE-117  |   VSS   GND
53   Pin_I/O   pin_name   A7   |   DM_n_DBI_n_TDQS_t  DM_DBI_TDQS
54   Pin_I/O   pin_name   C2   |   DQ0   DQ
55   Pin_I/O   pin_name   B7   |   DQ1   DQ
56   Pin_I/O   pin_name   D3   |   DQ2   DQ
57   Pin_I/O   pin_name   D7   |   DQ3   DQ
58   Pin_I/O   pin_name   D2   |   DQ4   DQ
59   Pin_I/O   pin_name   D8   |   DQ5   DQ
60   Pin_I/O   pin_name   E3   |   DQ6   DQ
61   Pin_I/O   pin_name   E7   |   DQ7   DQ
62   Pin_I/O   pin_name   B3   |   DQS_c   DQS
63   Pin_I/O   pin_name   C3   |   DQS_t   DQS
64   Pin_Rail   pin_name   A1   |   VDD   POWER
65   Pin_Rail   pin_name   B2   |   VDDQ   POWER
66   Pin_Rail   pin_name   B8   |   VDDQ   POWER
67   Pin_Rail   pin_name   A2   |   VSS   GND
[End Interconnect Model]
[Interconnect Model]   z11b_x8_ondie_PDN_iss
File_IBIS-ISS   z11b_x8_ondie_PDN.iss   z11b_x8_ondie_PDN
Number_of_terminals = 85
1   Pad_I/O   pin_name   A7   |   DM_n_DBI_n_TDQS_t  DM_DBI_TDQS
2   Pad_I/O   pin_name   C2   |   DQ0   DQ
3   Pad_I/O   pin_name   B7   |   DQ1   DQ
4   Pad_I/O   pin_name   D3   |   DQ2   DQ
5   Pad_I/O   pin_name   D7   |   DQ3   DQ
6   Pad_I/O   pin_name   D2   |   DQ4   DQ
7   Pad_I/O   pin_name   D8   |   DQ5   DQ
8   Pad_I/O   pin_name   E3   |   DQ6   DQ
9   Pad_I/O   pin_name   E7   |   DQ7   DQ
10   Pad_I/O   pin_name   B3   |   DQS_c   DQS
11   Pad_I/O   pin_name   C3   |   DQS_t   DQS
12   Pad_Rail   pad_name   VDDQ_DIE-4   |   VDDQ   POWER
13   Pad_Rail   pad_name   VDDQ_DIE-8   |   VDDQ   POWER
14   Pad_Rail   pad_name   VDDQ_DIE-13  |   VDDQ   POWER
15   Pad_Rail   pad_name   VDDQ_DIE-16  |   VDDQ   POWER
16   Pad_Rail   pad_name   VDDQ_DIE-20  |   VDDQ   POWER
17   Pad_Rail   pad_name   VDDQ_DIE-25  |   VDDQ   POWER
18   Pad_Rail   pad_name   VDDQ_DIE-36  |   VDDQ   POWER
19   Pad_Rail   pad_name   VDDQ_DIE-48  |   VDDQ   POWER
20   Pad_Rail   pad_name   VDDQ_DIE-52  |   VDDQ   POWER
21   Pad_Rail   pad_name   VDDQ_DIE-62  |   VDDQ   POWER
22   Pad_Rail   pad_name   VDDQ_DIE-40  |   VDDQ   POWER
23   Pad_Rail   pad_name   VDDQ_DIE-45  |   VDDQ   POWER
24   Pad_Rail   pad_name   VDDQ_DIE-57  |   VDDQ   POWER
25   Pad_Rail   pad_name   VSS_DIE-2   |   VSS   GND
26   Pad_Rail   pad_name   VSS_DIE-6   |   VSS   GND
27   Pad_Rail   pad_name   VSS_DIE-10   |   VSS   GND
28   Pad_Rail   pad_name   VSS_DIE-11   |   VSS   GND
29   Pad_Rail   pad_name   VSS_DIE-15   |   VSS   GND
30   Pad_Rail   pad_name   VSS_DIE-18   |   VSS   GND
31   Pad_Rail   pad_name   VSS_DIE-22   |   VSS   GND
32   Pad_Rail   pad_name   VSS_DIE-23   |   VSS   GND
33   Pad_Rail   pad_name   VSS_DIE-27   |   VSS   GND
34   Pad_Rail   pad_name   VSS_DIE-28   |   VSS   GND
35   Pad_Rail   pad_name   VSS_DIE-32   |   VSS   GND
36   Pad_Rail   pad_name   VSS_DIE-34   |   VSS   GND
37   Pad_Rail   pad_name   VSS_DIE-38   |   VSS   GND
38   Pad_Rail   pad_name   VSS_DIE-42   |   VSS   GND
39   Pad_Rail   pad_name   VSS_DIE-43   |   VSS   GND
40   Pad_Rail   pad_name   VSS_DIE-47   |   VSS   GND
41   Pad_Rail   pad_name   VSS_DIE-50   |   VSS   GND
42   Pad_Rail   pad_name   VSS_DIE-54   |   VSS   GND
43   Pad_Rail   pad_name   VSS_DIE-55   |   VSS   GND
44   Pad_Rail   pad_name   VSS_DIE-59   |   VSS   GND
45   Pad_Rail   pad_name   VSS_DIE-60   |   VSS   GND
46   Pad_Rail   pad_name   VSS_DIE-64   |   VSS   GND
47   Pad_Rail   pad_name   VSS_DIE-66   |   VSS   GND
48   Pad_Rail   pad_name   VSS_DIE-69   |   VSS   GND
49   Pad_Rail   pad_name   VSS_DIE-72   |   VSS   GND
50   Pad_Rail   pad_name   VSS_DIE-93   |   VSS   GND
51   Pad_Rail   pad_name   VSS_DIE-109  |   VSS   GND
52   Pad_Rail   pad_name   VSS_DIE-117  |   VSS   GND
53   Buffer_I/O   pin_name   A7   |   DM_n_DBI_n_TDQS_t  DM_DBI_TDQS
54   Pulldown_ref   pin_name   A7   |   DM_n_DBI_n_TDQS_t  DM_DBI_TDQS
55   Pullup_ref   pin_name   A7   |   DM_n_DBI_n_TDQS_t  DM_DBI_TDQS
56   Buffer_I/O   pin_name   C2   |   DQ0   DQ
57   Pulldown_ref   pin_name   C2   |   DQ0   DQ
58   Pullup_ref   pin_name   C2   |   DQ0   DQ
59   Buffer_I/O   pin_name   B7   |   DQ1   DQ
60   Pulldown_ref   pin_name   B7   |   DQ1   DQ
61   Pullup_ref   pin_name   B7   |   DQ1   DQ
62   Buffer_I/O   pin_name   D3   |   DQ2   DQ
63   Pulldown_ref   pin_name   D3   |   DQ2   DQ
64   Pullup_ref   pin_name   D3   |   DQ2   DQ
65   Buffer_I/O   pin_name   D7   |   DQ3   DQ
66   Pulldown_ref   pin_name   D7   |   DQ3   DQ
67   Pullup_ref   pin_name   D7   |   DQ3   DQ
68   Buffer_I/O   pin_name   D2   |   DQ4   DQ
69   Pulldown_ref   pin_name   D2   |   DQ4   DQ
70   Pullup_ref   pin_name   D2   |   DQ4   DQ
71   Buffer_I/O   pin_name   D8   |   DQ5   DQ
72   Pulldown_ref   pin_name   D8   |   DQ5   DQ
73   Pullup_ref   pin_name   D8   |   DQ5   DQ
74   Buffer_I/O   pin_name   E3   |   DQ6   DQ
75   Pulldown_ref   pin_name   E3   |   DQ6   DQ
76   Pullup_ref   pin_name   E3   |   DQ6   DQ
77   Buffer_I/O   pin_name   E7   |   DQ7   DQ
78   Pulldown_ref   pin_name   E7   |   DQ7   DQ
79   Pullup_ref   pin_name   E7   |   DQ7   DQ
80   Buffer_I/O   pin_name   B3   |   DQS_c   DQS
81   Pulldown_ref   pin_name   B3   |   DQS_c   DQS
82   Pullup_ref   pin_name   B3   |   DQS_c   DQS
83   Buffer_I/O   pin_name   C3   |   DQS_t   DQS
84   Pulldown_ref   pin_name   C3   |   DQS_t   DQS
85   Pullup_ref   pin_name   C3   |   DQS_t   DQS
[End Interconnect Model]
[End Interconnect Model Set]
| Interconnect Model Set for MT40A1G8SA_DQ_Uncoupled_Sparam
[Interconnect Model Set]   MT40A1G8SA_DQ_Uncoupled_Sparam
[Interconnect Model]   z11b_78b_dm_sparam_s2p
File_TS   z11b_78b_dm_sparam.s2p
Number_of_terminals = 3
1   Buffer_I/O   pin_name   A7   |   DM_n_DBI_n_TDQS_t  DM_DBI_TDQS
2   Pin_I/O   pin_name   A7   |   DM_n_DBI_n_TDQS_t  DM_DBI_TDQS
3   Pin_Rail   signal_name   VSS   |   VSS   GND
[End Interconnect Model]
[Interconnect Model]   z11b_78b_dq0_sparam_s2p
File_TS   z11b_78b_dq0_sparam.s2p
Number_of_terminals = 3
1   Buffer_I/O   pin_name   C2   |   DQ0   DQ
2   Pin_I/O   pin_name   C2   |   DQ0   DQ
3   Pin_Rail   signal_name   VSS   |   VSS   GND
[End Interconnect Model]
[Interconnect Model]   z11b_78b_dq1_sparam_s2p
File_TS   z11b_78b_dq1_sparam.s2p
Number_of_terminals = 3
1   Buffer_I/O   pin_name   B7   |   DQ1   DQ
2   Pin_I/O   pin_name   B7   |   DQ1   DQ
3   Pin_Rail   signal_name   VSS   |   VSS   GND
[End Interconnect Model]
[Interconnect Model]   z11b_78b_dq2_sparam_s2p
File_TS   z11b_78b_dq2_sparam.s2p
Number_of_terminals = 3
1   Buffer_I/O   pin_name   D3   |   DQ2   DQ
2   Pin_I/O   pin_name   D3   |   DQ2   DQ
3   Pin_Rail   signal_name   VSS   |   VSS   GND
[End Interconnect Model]
[Interconnect Model]   z11b_78b_dq3_sparam_s2p
File_TS   z11b_78b_dq3_sparam.s2p
Number_of_terminals = 3
1   Buffer_I/O   pin_name   D7   |   DQ3   DQ
2   Pin_I/O   pin_name   D7   |   DQ3   DQ
3   Pin_Rail   signal_name   VSS   |   VSS   GND
[End Interconnect Model]
[Interconnect Model]   z11b_78b_dq4_sparam_s2p
File_TS   z11b_78b_dq4_sparam.s2p
Number_of_terminals = 3
1   Buffer_I/O   pin_name   D2   |   DQ4   DQ
2   Pin_I/O   pin_name   D2   |   DQ4   DQ
3   Pin_Rail   signal_name   VSS   |   VSS   GND
[End Interconnect Model]
[Interconnect Model]   z11b_78b_dq5_sparam_s2p
File_TS   z11b_78b_dq5_sparam.s2p
Number_of_terminals = 3
1   Buffer_I/O   pin_name   D8   |   DQ5   DQ
2   Pin_I/O   pin_name   D8   |   DQ5   DQ
3   Pin_Rail   signal_name   VSS   |   VSS   GND
[End Interconnect Model]
[Interconnect Model]   z11b_78b_dq6_sparam_s2p
File_TS   z11b_78b_dq6_sparam.s2p
Number_of_terminals = 3
1   Buffer_I/O   pin_name   E3   |   DQ6   DQ
2   Pin_I/O   pin_name   E3   |   DQ6   DQ
3   Pin_Rail   signal_name   VSS   |   VSS   GND
[End Interconnect Model]
[Interconnect Model]   z11b_78b_dq7_sparam_s2p
File_TS   z11b_78b_dq7_sparam.s2p
Number_of_terminals = 3
1   Buffer_I/O   pin_name   E7   |   DQ7   DQ
2   Pin_I/O   pin_name   E7   |   DQ7   DQ
3   Pin_Rail   signal_name   VSS   |   VSS   GND
[End Interconnect Model]
[Interconnect Model]   z11b_78b_dq0_sparam_s2p
File_TS   z11b_78b_dqs_sparam.s4p
Number_of_terminals = 5
1   Buffer_I/O   pin_name   B3   |   DQS_c   DQS
2   Pin_I/O   pin_name   B3   |   DQS_c   DQS
3   Buffer_I/O   pin_name   C3   |   DQS_t   DQS
4   Pin_I/O   pin_name   C3   |   DQS_t   DQS
5   Pin_Rail   signal_name   VSS   |   VSS   GND
[End Interconnect Model]
[Interconnect Model]   z11b_78b_tdqs_sparam_s2p
File_TS   z11b_78b_tdqs_sparam.s2p
Number_of_terminals = 3
1   Buffer_I/O   pin_name   A3   |   TDQS_c   TDQS
2   Pin_I/O   pin_name   A3   |   TDQS_c   TDQS
3   Pin_Rail   signal_name   VSS   |   VSS   GND
[End Interconnect Model]
[End Interconnect Model Set]
| Models and submodels in the file (52): DQ_34_3200 (I/O), DQ_40_3200 (I/O), DQ_48_3200 (I/O), DQ_IN_ODTOFF_3200 (Input), DQ_IN_ODT34_3200 (Input), DQ_IN_ODT40_3200 (Input), DQ_IN_ODT48_3200 (Input), DQ_IN_ODT60_3200 (Input), DQ_IN_ODT80_3200 (Input), DQ_IN_ODT120_3200 (Input), DQ_IN_ODT240_3200 (Input), DQS_34_3200 (I/O), DQS_40_3200 (I/O), DQS_48_3200 (I/O), DQS_IN_ODTOFF_3200 (Input), DQS_IN_ODT34_3200 (Input), DQS_IN_ODT40_3200 (Input), DQS_IN_ODT48_3200 (Input), DQS_IN_ODT60_3200 (Input), DQS_IN_ODT80_3200 (Input), DQS_IN_ODT120_3200 (Input), DQS_IN_ODT240_3200 (Input), DM_ODTOFF_3200 (Input), DM_ODT34_3200 (Input), DM_ODT40_3200 (Input), DM_ODT48_3200 (Input), DM_ODT60_3200 (Input), DM_ODT80_3200 (Input), DM_ODT120_3200 (Input), DM_ODT240_3200 (Input), TDQS_ODTOFF_3200 (Terminator), TDQS_ODT34_3200 (Terminator), TDQS_ODT40_3200 (Terminator), TDQS_ODT48_3200 (Terminator), TDQS_ODT60_3200 (Terminator), TDQS_ODT80_3200 (Terminator), TDQS_ODT120_3200 (Terminator), TDQS_ODT240_3200 (Terminator), INPUT (Input), CLKIN (Input), RESET (Input), TEN (Input), ALERT (Open_sink), NF_DQ (Terminator), NF_INPUT (Terminator), 34ohm_ODT_3200 (Dynamic_clamp), 40ohm_ODT_3200 (Dynamic_clamp), 48ohm_ODT_3200 (Dynamic_clamp), 60ohm_ODT_3200 (Dynamic_clamp), 80ohm_ODT_3200 (Dynamic_clamp), 120ohm_ODT_3200 (Dynamic_clamp), 240ohm_ODT_3200 (Dynamic_clamp)
